FUNCTION_BLOCK Valve
VAR_INPUT
	bValveEnable_In		: BOOL;
	bInterlock1_In		: BOOL;
	bInterlock2_In		: BOOL;
	bInterlock3_In		: BOOL;
	bInterlock4_In		: BOOL;
	bInterlock5_In		: BOOL;
	bValveInterlock_In	: BOOL;
	bPMCCtrl_In			: BOOL;
	bForceOpen_In		: BOOL;
END_VAR
VAR_OUTPUT
	bValveOpen_Out		: BOOL;
END_VAR
VAR
END_VAR

IF bValveEnable_In THEN
	IF bInterlock1_In AND bInterlock2_In AND bInterlock3_In AND bInterlock4_In AND bInterlock5_In THEN
		IF bForceOpen_In OR ( bValveInterlock_In AND bPMCCtrl_In ) THEN
			bValveOpen_Out := TRUE ;
		ELSE
			bValveOpen_Out := FALSE ;
		END_IF
	ELSE
			bValveOpen_Out := FALSE ;
	END_IF
END_IF

END_FUNCTION_BLOCK
